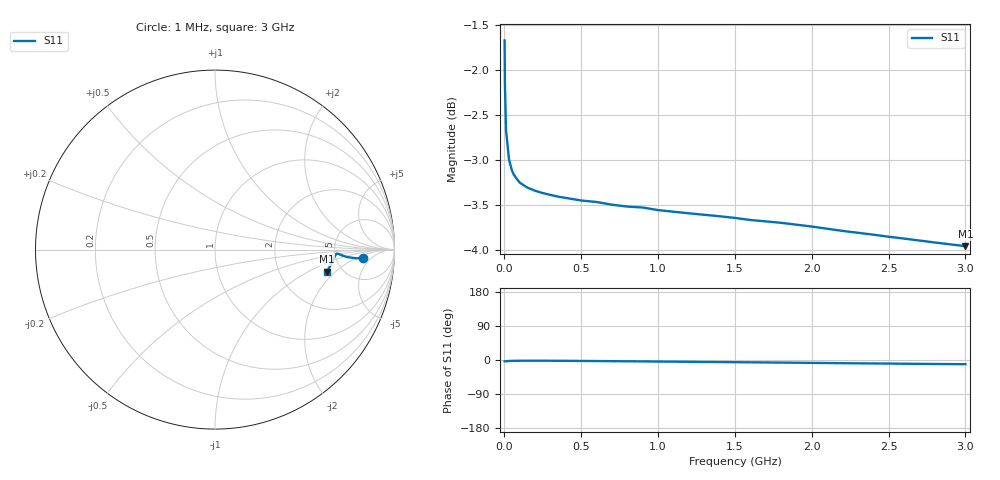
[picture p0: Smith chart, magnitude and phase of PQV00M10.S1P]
! SIEMENS Small Signal Semiconductors
! BAR64-04
! Si PIN Diode in SOT23 (2 diodes in series, pin 3 open)
! IF = 0.1 mA
! S-Parameters:  July  1992
# GHz  S  MA  R  50
!  f  S11
! GHz  MAG  ANG
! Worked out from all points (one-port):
!   33 points, 1 MHz to 3 GHz, reference 50 ohm
!   lowest |S11| = -4.0 dB at 3 GHz (marker M1), VSWR 4.47, Z = 190 - j77.5 ohm
!   |S11| at or under -10 dB: nowhere
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0.001  0.8248 -3.4
0.003  0.7812 -3.5
0.01  0.7357 -3.2
0.03  0.708 -2.6
0.05  0.6981 -2.3
0.06  0.6951 -2.2
0.1  0.6878 -2.0
0.15  0.6834 -1.9
0.25  0.6787 -1.9
0.4  0.6745 -2.2
0.45  0.6734 -2.3
0.5  0.6723 -2.5
0.6  0.671 -2.8
0.8  0.6671 -3.4
0.9  0.6663 -3.7
1  0.6641 -4.1
1.2  0.6614 -4.7
1.4  0.6589 -5.4
1.5  0.6575 -5.8
1.6  0.6558 -6.1
1.8  0.6534 -6.8
2  0.6503 -7.6
2.2  0.6467 -8.4
2.4  0.6436 -9.1
2.5  0.6419 -9.4
2.6  0.6404 -9.8
2.8  0.6372 -10.5
3  0.6342 -11.1
